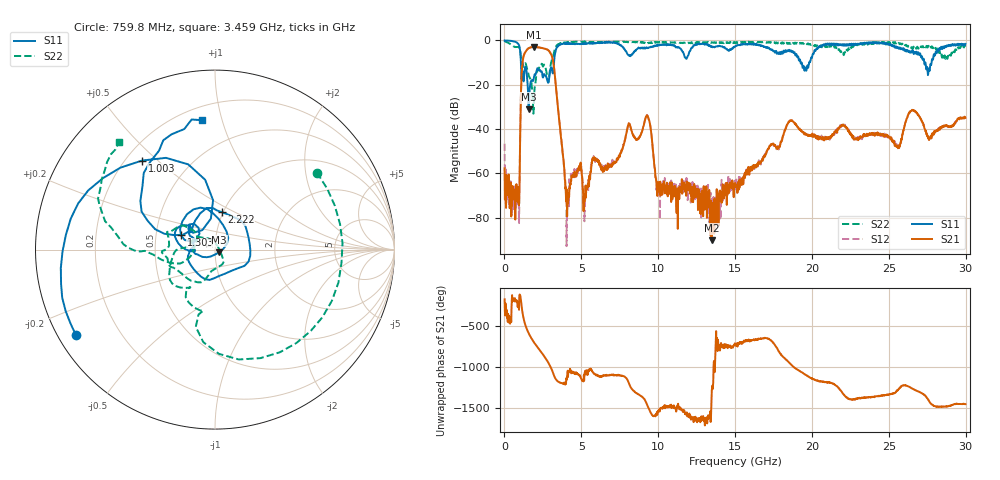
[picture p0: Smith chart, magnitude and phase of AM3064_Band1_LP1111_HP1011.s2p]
# Hz S DB R 50.0
!freq dBS11 angS11 dBS21 angS21 dBS12 angS12 dBS22 angS22
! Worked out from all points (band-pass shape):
!   1600 points, 10 MHz to 29.98 GHz, reference 50 ohm
!   highest |S21| = -2.94 dB at 1.941 GHz (marker M1); lowest = -90.2 dB at 13.47 GHz (marker M2)
!   |S21| within 3 dB of the highest: 1.306 GHz to 3.01 GHz (1.704 GHz wide, 78.9 % of centre)
!   lowest |S11| = -31.1 dB at 1.566 GHz (marker M3), VSWR 1.06, Z = 52.4 - j1.6 ohm
!   |S11| at or under -10 dB: 1.071 GHz to 3.222 GHz (2.151 GHz wide, 100 % of centre); 19.26 GHz to 19.82 GHz (562.6 MHz wide, 2.88 % of centre); 27.38 GHz to 27.78 GHz (404.7 MHz wide, 1.47 % of centre)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
!   |S22| runs from -33.1 to -0.2 dB; largest |S21 - S12| = 0.012
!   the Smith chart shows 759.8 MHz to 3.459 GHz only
!   S11 on the Smith chart (normalised r, x): 759.8 MHz: 0.05, -0.28; 1.003 GHz: 0.26, +0.45; 1.303 GHz: 0.67, +0.11; 2.222 GHz: 0.98, +0.43; 3.459 GHz: 0.28, +0.86
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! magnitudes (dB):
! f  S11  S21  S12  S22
! 10 MHz  -0.1  -57.7  -46.6  -0.2
! 759.8 MHz  -0.8  -69.2  -70.8  -3.0
! 1.003 GHz  -3.9  -51.2  -51.3  -4.1
! 1.303 GHz  -13.7  -6.0  -5.9  -11.2
! 1.566 GHz  -31.1  -3.6  -3.5  -15.5
! 1.941 GHz  -16.0  -2.9  -2.9  -23.7
! 2.222 GHz  -13.5  -3.2  -3.1  -12.8
! 3.046 GHz  -12.3  -6.4  -6.4  -9.7
! 3.459 GHz  -2.8  -28.9  -29.0  -1.9
! 4.04 GHz  -1.6  -67.2  -92.9  -0.9
! 5.015 GHz  -1.4  -58.6  -58.7  -0.5
! 5.277 GHz  -1.5  -65.5  -69.0  -0.6
! 9.269 GHz  -3.2  -34.1  -33.6  -1.2
! 10 GHz  -2.2  -66.5  -67.2  -0.9
! 13.47 GHz  -2.7  -90.2  -71.8  -0.9
! 15 GHz  -2.8  -64.3  -64.1  -1.2
! 18.57 GHz  -5.0  -36.3  -36.1  -1.3
! 19.99 GHz  -8.0  -43.2  -43.4  -1.8
! 25 GHz  -1.5  -43.7  -43.5  -1.0
! 26.55 GHz  -4.5  -31.4  -31.5  -3.9
! 27.56 GHz  -15.2  -44.1  -44.1  -2.6
! 29.98 GHz  -1.6  -34.9  -35.0  -2.8
